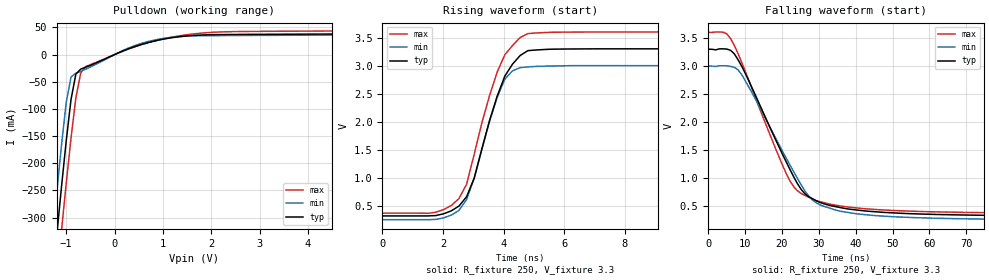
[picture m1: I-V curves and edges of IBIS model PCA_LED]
| PCA9553 Ibis Model from Interface Products of Philips Semiconductors
| 4-bit I2c LED driver with programmable blink rates
|   Available in tssop8 and so8 packages.
[IBIS Ver]   3.2
[Comment Char]   |_char
[File name]   pca9553_3v.ibs
[File Rev]   1.0
[Date]   Mar 18, 2004
[Source]
Generated from ITK by TGA Tempe
[Notes]
   From the pca9551.hsp file.
[Disclaimer]
Philips Semiconductors warrants and represents that the IBIS models
identified herein are owned by Philips Semiconductors (PHILIPS). The models
provided are not warranted as fully representing all of the operating
characteristics and specifications of the semiconductor products to which the
models relate. Moreover, unless there is a signed, written agreement to the
contrary, these models are furnished on an "as is" basis without support or
warranty of any kind, either expressed or implied, regarding the use thereof,
and PHILIPS specifically disclaims all implied warranties of merchantability
and fitness of the models for any purpose. PHILIPS does not assume any
liability arising out of the application or use of these IBIS models including
infringement of patents and copyrights, nor does PHILIPS convey any license
under its patents and copyrights or the rights of others. PHILIPS provides
SPICE models as a service to our customers. You and your company shall not
distribute, convey, sell, or give these models to anyone else without
receiving prior written permission from PHILIPS. PHILIPS reserves the right
to make changes without notice to these IBIS models to improve reliability,
function, or design.
[Copyright]
Copyright 2004, Philips Semiconductors, All rights reserved.
[Component]   PCA9553DP01
Si_location Pin
Timing_location Pin
[Manufacturer]   Philips Semiconductors
[Package]
R_pkg   34m   30m   37m
L_pkg   1.74n   1.67n   1.81n
C_pkg   0.5p   0.5p   0.5p
| TSSOP8 package
[Pin] signal_name   model_name   R_pin   L_pin   C_pin
1   LED0   PCA_LED   37m   1.81n   0.5p
2   LED0   PCA_LED   30m   1.67n   0.5p
3   LED0   PCA_LED   30m   1.67n   0.5p
4   VSS   GND   37m   1.81n   0.5p
5   LED0   PCA_LED   37m   1.81n   0.5p
6   SCL   PCA_IN   30m   1.67n   0.5p
7   SDA   PCA_IN   30m   1.67n   0.5p
8   VDD   POWER   37m   1.81n   0.5p
[Component]   PCA9553D01
Si_location Pin
Timing_location Pin
[Manufacturer]   Philips Semiconductors
[Package]
R_pkg   49m   36m   62m
L_pkg   4.45n   4.03n   4.87n
C_pkg   0.5p   0.5p   0.5p
| SO8 package
[Pin] signal_name   model_name   R_pin   L_pin   C_pin
1   LED0   PCA_LED   62m   4.87n   0.5p
2   LED0   PCA_LED   36m   4.03n   0.5p
3   LED0   PCA_LED   36m   4.03n   0.5p
4   VSS   GND   62m   4.87n   0.5p
5   LED0   PCA_LED   62m   4.87n   0.5p
6   SCL   PCA_IN   36m   4.03n   0.5p
7   SDA   PCA_IN   36m   4.03n   0.5p
8   VDD   POWER   62m   4.88n   0.5p
[Model]   PCA_IN
Model_type Input
Vinh=3.0
Vinl=0
C_comp   0.5p   0.5p   0.5p
[Temperature Range] 25   -40   85
[Voltage Range]   3.3   3.0   3.6
[Pullup Reference]  3.3   3.0   3.6
[Pulldown Reference]0   0   0
[POWER Clamp Reference]3.3   3.0   3.6
[GND Clamp Reference]0   0   0
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| Models and submodels in the file (2): PCA_IN (Input), PCA_LED (Open_drain)
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[Model]   PCA_LED
Model_type Open_drain
C_comp   0.5p   0.5p   0.5p
[Model Spec]
[Temperature Range] 25   -40   85
[Voltage Range]   3.3   3.0   3.6
[Pullup Reference]  3.3   3.0   3.6
[Pulldown Reference]0   0   0
[POWER Clamp Reference]3.3   3.0   3.6
[GND Clamp Reference]0   0   0
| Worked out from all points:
|   slope of the pulldown table from 0 to 0.495 V, typ, clamps not added: 29 ohm
|   falling waveform, R_fixture 250, V_fixture 3.3: 20-80 % time 12.8ns typ, 13.4ns min, 11.9ns max; typ from 3.3 V to 0.33 V
|   rising waveform, R_fixture 250, V_fixture 3.3: 20-80 % time 992ps typ, 895ps min, 1ns max; typ from 0.325 V to 3.3 V
[Pulldown]
-3.3V     -2.384A    -2.312A    -2.462A
-1.3V     -430.1mA   -351.5mA   -511.9mA
-1.2V     -336.9mA   -258.7mA   -418.5mA
-1.1V     -246mA     -169.2mA   -326.7mA
-1V       -159.3mA   -88.52mA   -237.6mA
-900mV    -82.59mA   -41.02mA   -153.4mA
-800mV    -35.93mA   -34.24mA   -79.86mA
-700mV    -26.7mA    -30.83mA   -33.95mA
300mV     11.09mA    12.53mA    10.57mA
1V        28.33mA    29.75mA    28.72mA
2V        36.6mA     34.92mA    40.93mA
6.6V      41.65mA    40.69mA    46.63mA
[Falling Waveform]
R_fixture=250
V_fixture=3.3
V_fixture_min=3.0
V_fixture_max=3.6
0s        3.3V       3V         3.6V
5.051ns   3.303V     3.006V     3.574V
8.081ns   3.116V     2.934V     3.225V
12.12ns   2.58V      2.497V     2.556V
21.21ns   1.286V     1.354V     1.08V
23.23ns   1.022V     1.113V     847.2mV
26.26ns   724.1mV    773.6mV    695.5mV
30.3ns    570.7mV    527.9mV    583.9mV
41.41ns   426.5mV    359.6mV    464.8mV
100ns     329.8mV    262.7mV    378.3mV
[Rising Waveform]
R_fixture=250
V_fixture=3.3
V_fixture_min=3.0
V_fixture_max=3.6
0s        324.7mV    257.7mV    373.8mV
1.768ns   331.5mV    263.2mV    391.3mV
2.525ns   499.5mV    422.4mV    633mV
2.778ns   665.8mV    615.1mV    886.5mV
3.03ns    998.4mV    995.8mV    1.423V
3.535ns   2.02V      2.011V     2.467V
4.04ns    2.815V     2.759V     3.195V
4.293ns   3.027V     2.908V     3.359V
4.798ns   3.267V     2.977V     3.571V
25ns      3.3V       3V         3.6V
[Ramp]
R_load=250
dV/dt_r   1.785E+0/9.646E-10   1.645E+0/8.874E-10   1.936E+0/9.986E-10
dV/dt_f   1.501E+0/1.049E-8   1.261E+0/9.980E-9   1.722E+0/1.031E-8
|[End   PCA_LED
